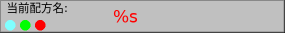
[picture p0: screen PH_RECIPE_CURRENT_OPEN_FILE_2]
VISUALIZATION PH_RECIPE_CURRENT_OPEN_FILE_2  // 285x33
VAR_INPUT
	RECIPE_CTRL_V2 : ST_RecipeCtrl_2;
END_VAR
VAR_INPUT
	Right_Edge_Rel : UDINT;
END_VAR
    Rectangle (0,0 285x33), "当前配方名:", text list: 'TextList_Recipe', text index: 101
        p874137650: Right_Edge_Rel
    Rectangle (110,0 175x33), "%s", text variable: RECIPE_CTRL_V2.sStatus.sgCurUsedFileDisplay
        p874137650: Right_Edge_Rel
    Ellipse (5,20 10x10), colour toggle: (RECIPE_CTRL_V2.sStatus.bFlashLamp) <> 0, invisible if: NOT RECIPE_CTRL_V2.sStatus.bBusy
    Ellipse (20,20 10x10), invisible if: NOT RECIPE_CTRL_V2.sStatus.bDone
    Ellipse (35,20 10x10), invisible if: NOT RECIPE_CTRL_V2.sStatus.bError
END_VISUALIZATION
